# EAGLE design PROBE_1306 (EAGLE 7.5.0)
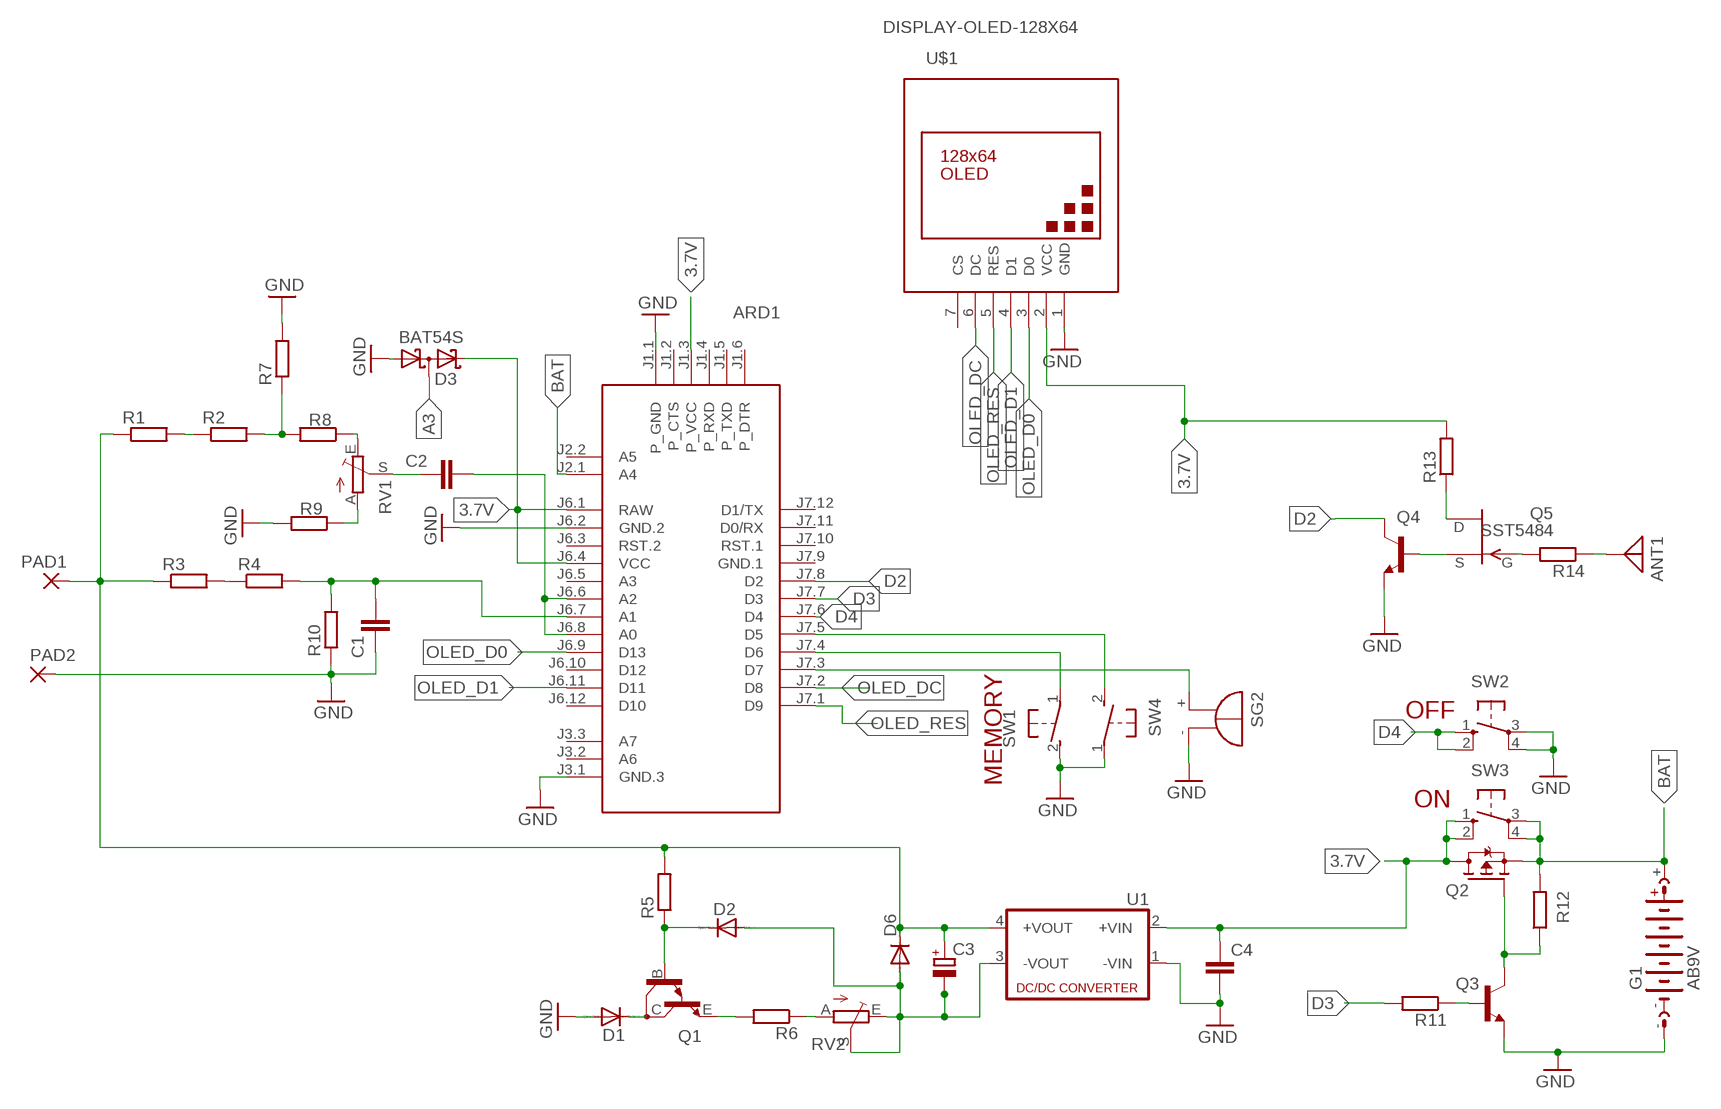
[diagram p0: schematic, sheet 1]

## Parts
ANT1  ANTENNA  [PAD-01]
ARD1  ARDUINO-PRO-MINI-3.3V  [ARDUINO-PRO-MINI]
C1  C-EUC1206  [C1206]
C2  C-EUC1206  [C1206]
C3  CPOL-EUC/6032-28R  [C/6032-28R]
C4  C-EUC1206  [C1206]
D1  CGRM4007-G  [SOD-123_MINI-SMA]
D2  CGRM4007-G  [SOD-123_MINI-SMA]
D3  BAT54S  [SOT23]
D6  CGRM4001-G  [SOD-123_MINI-SMA]
G1  AB9V  [AB9V]
PAD1  3,81/1,1  [3,81/1,1]
PAD2  3,81/1,1  [3,81/1,1]
Q1  BDV65  [SOT93]
Q2  STR2P3LLH6  [SOT23]
Q3  BC817-16LT1SMD  [SOT23-BEC]
Q4  BC817-16LT1SMD  [SOT23-BEC]
Q5  SST5484  [SOT23]
R1  R-EU_R2512  [R2512]
R2  R-EU_R2512  [R2512]
R3  R-EU_R2512  [R2512]
R4  R-EU_R2512  [R2512]
R5  R-EU_R2512  [R2512]
R6  R-EU_R2512  [R2512]
R7  R-EU_R2512  [R2512]
R8  R-EU_R0805  [R0805]
R9  R-EU_R0805  [R0805]
R10  R-EU_R2512  [R2512]
R11  R-EU_R0805  [R0805]
R12  R-EU_R0805  [R0805]
R13  R-EU_R0805  [R0805]
R14  R-EU_R0805  [R0805]
RV1  TRIM_EU-CT6  [CT6]
RV2  TRIM_EU-CT6  [CT6]
SG2  BMT1205XH7.5  [BMT1205XH7.5]
SW1  31-XX  [B3F-31XX]
SW2  10-XX  [B3F-10XX]
SW3  10-XX  [B3F-10XX]
SW4  31-XX  [B3F-31XX]
U1  NME  [NME]
U$1  DISPLAY-OLED-128X64  [DISPLAY-OLED-128X64]

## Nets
3.7V: ARD1.J1.3(P_VCC) ARD1.J6.1(RAW) ARD1.J6.4(VCC) C4.1 D3.2(C2) Q2.1(D) R13.2 SW3.1(S) SW3.2(S1) U1.2(+VIN) U$1.2(VCC)
A3: ARD1.J6.7(A1) C1.2 D3.3(C1A2) R4.2 R10.2
BAT: ARD1.J2.1(A4) G1.+ Q2.3(S) R12.2 SW3.3(P) SW3.4(P1)
D2: ARD1.J7.8(D2) Q4.C
D3: ARD1.J7.7(D3) R11.2
D4: ARD1.J7.6(D4) SW2.1(S) SW2.2(S1)
GND: ARD1.J1.1(P_GND) ARD1.J3.1(GND.3) ARD1.J6.2(GND.2) C1.1 C4.2 D1.A D3.1(A1) G1.- PAD2.1(P) Q3.E Q4.E R7.2 R9.2 R10.1 SG2.- SW1.2(S) SW2.3(P) SW2.4(P1) SW4.1(P) U1.1(-VIN) U$1.1(GND)
N$1: R2.2 R7.1 R8.2
N$2: R8.1 RV1.E
N$3: R9.1 RV1.A
N$4: ARD1.J6.6(A2) ARD1.J6.8(A0) C2.2
N$5: ANT1.1 R14.1
N$6: ARD1.J7.5(D5) SW4.2(S)
N$7: Q4.B Q5.3(S)
N$8: Q1.E R6.2
N$9: R6.1 RV2.A
N$10: C3.- D2.A D6.A RV2.E RV2.S U1.3(-VOUT)
N$11: ARD1.J7.4(D6) SW1.1(P)
N$12: D1.C Q1.C
N$13: Q5.1(G) R14.2
N$14: Q5.2(D) R13.1
N$15: ARD1.J7.3(D7) SG2.+
N$16: Q2.2(G) Q3.C R12.1
N$17: C3.+ D6.C PAD1.1(P) R1.1 R3.1 R5.2 U1.4(+VOUT)
N$18: Q3.B R11.1
N$20: D2.C Q1.B R5.1
N$23: C2.1 RV1.S
N$24: R1.2 R2.1
N$26: R3.2 R4.1
OLED_D0: ARD1.J6.9(D13) U$1.3(D0)
OLED_D1: ARD1.J6.11(D11) U$1.4(D1)
OLED_DC: ARD1.J7.2(D8) U$1.6(DC)
OLED_RES: ARD1.J7.1(D9) U$1.5(RES)
Unconnected: ARD1.J1.2(P_CTS) ARD1.J1.4(P_RXD) ARD1.J1.5(P_TXD) ARD1.J1.6(P_DTR) ARD1.J2.2(A5) ARD1.J3.2(A6) ARD1.J3.3(A7) ARD1.J6.3(RST.2) ARD1.J6.5(A3) ARD1.J6.10(D12) ARD1.J6.12(D10) ARD1.J7.10(RST.1) ARD1.J7.11(D0/RX) ARD1.J7.12(D1/TX) U$1.7(CS)

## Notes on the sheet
- OFF
- MEMORY
- ON

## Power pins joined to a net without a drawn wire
GND.1: ARD1.J7.9(GND.1)

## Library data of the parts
ANT1 = discrete:ANTENNA: Antenna
ARD1 = diy-modules:ARDUINO-PRO-MINI-*: Arduino Pro Mini and compatible devices More details available here: https://www.arduino.cc/en/Main/ArduinoBoardProMini Click here to find device on ebay.com
C1 C2 C4 = rcl:C-EU: CAPACITOR, European symbol
C3 = rcl:CPOL-EU: POLARIZED CAPACITOR, European symbol
D1 D2 D6 = diode:CGRM400*-G: Molded plasitc,JEDEC SOD-123/Mini SMA
D3 = diode:BAT54S: Schottky Diodes Pin connection corrected 2011-05-04 Source: Fairchild .. BAT54.pdf
G1 = battery:AB9V: 9-V BATTERY CLIP
PAD1 PAD2 = wirepad:3,81/1,1: THROUGH-HOLE PAD
Q1 = transistor:BDV65: NPN BIPOLAR DARLINGTON TRANSISTOR
Q2 = transistor-fet:STR2P3LLH6
Q3 Q4 = transistor-npn:BC817*: NPN Transistor
Q5 = transistor-fet:?548*: N-Channel JFETs Source: VISHAY 2N5484.pdf Compatible: TO92 2N5245 J304 J305 U310 J308 J309 J310 TO72 2N4416 2N4416A 2N3823 2N4351 3N169 3N170 3N171 MFE3002 TO18 2N3796 2N3797 MFE825 Source: Motorola European Master Guide Pacge 3-59
R1-R14 = rcl:R-EU_: RESISTOR, European symbol
RV1 RV2 = pot:TRIM_EU-: POTENTIOMETER
SG2 = buzzer:BMT1205XH7.5: MAGNETIC TRANSDUCER; OC_FARNELL: unknown; OC_NEWARK: unknown
SW1 SW4 = switch-omron:31-XX: OMRON SWITCH; MPN: B3F-3100; OC_FARNELL: 959704; OC_NEWARK: 36M3582
SW2 SW3 = switch-omron:10-XX: OMRON SWITCH; MPN: B3F-1000; OC_FARNELL: 176432; OC_NEWARK: 36M3542
U1 = dc-dc-converter:NME: DC-DC CONVERTER; MF: C & D TECHNOLOGIES, INC; MPN: NME1205D; OC_FARNELL: 1021466; OC_NEWARK: 98B8198
U$1 = diy-modules:DISPLAY-OLED-128X64: 128x64 Dot Matrix OLED Module based on SSD1306 chip Variant with SPI interface More details available here: http://www.instructables.com/id/How-to-use-OLED-display-arduino-module/ SSD1306 datasheet: https://cdn-shop.adafruit.com/datasheets/SSD1306.pdf Click here to find device on ebay.com Note: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

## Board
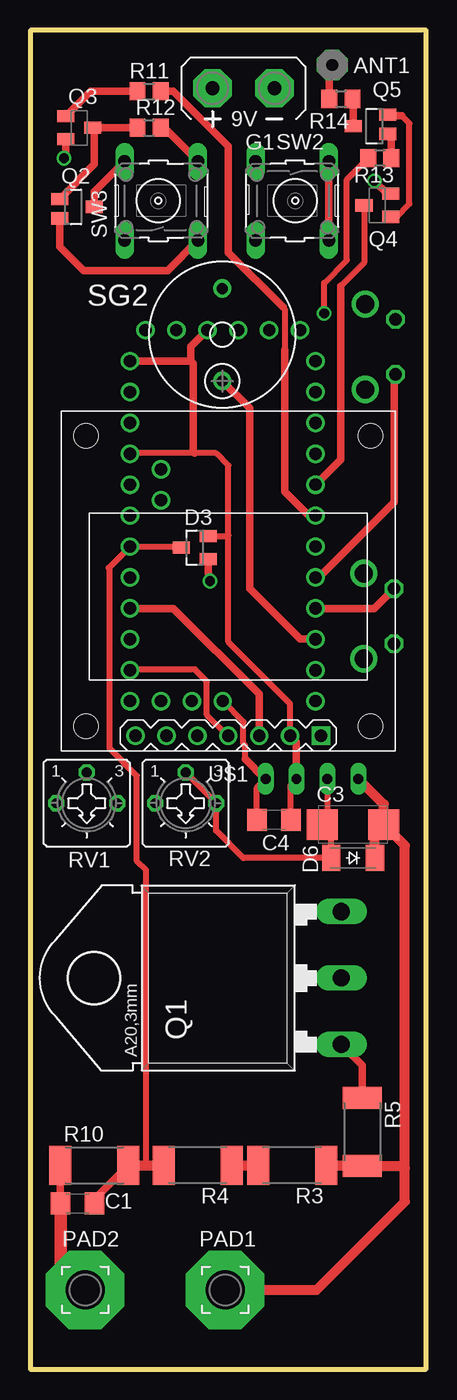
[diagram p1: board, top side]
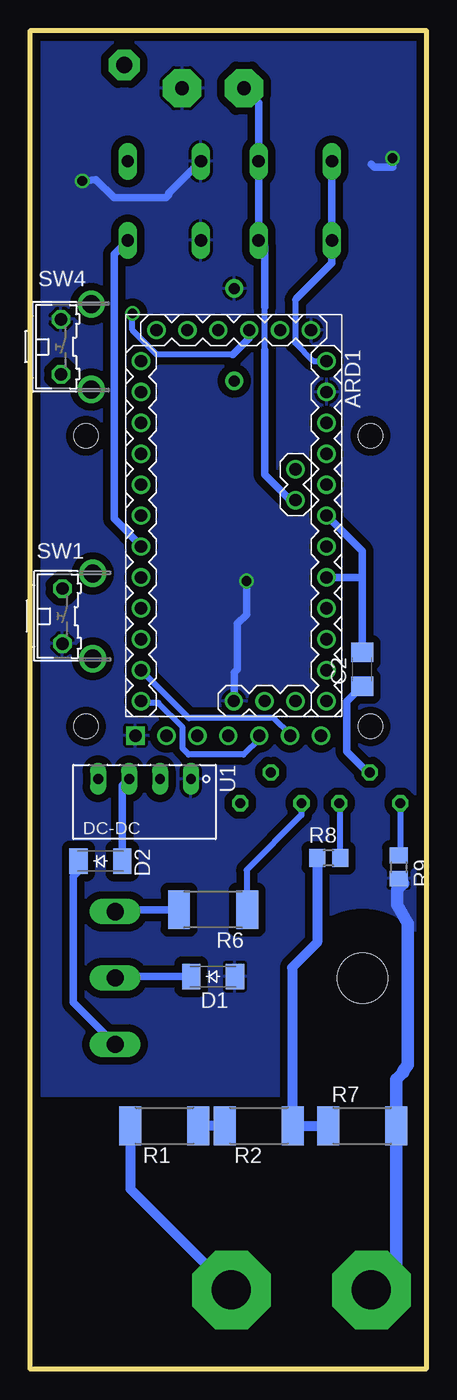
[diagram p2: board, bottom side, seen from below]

Size 32.5 x 110 mm. Coordinates in mm from the lower left corner, seen from the top.
Outline: 0,0 32.5,0 32.5,110 0,110 0,0
Copper layers (1*16): Top 0.035mm / dielectric 1.5mm / Bottom 0.035mm
Design rules "default *": minimum track width 10mil, minimum drill 24mil, track to track 8mil, track to pad 8mil, pad to pad 8mil, via to via 8mil, smd to smd 8mil, copper to edge 20mil, drill to drill 8mil, minimum pad ring 10mil, minimum via ring 8mil, stop-mask expansion 4mil, vias tented up to drill 0mil, thermal gap 10mil
bRestrict: area 0.4,22.6 to 10,28.2

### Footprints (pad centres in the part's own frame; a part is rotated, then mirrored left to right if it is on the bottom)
PAD-01 = drill 1.321 pad 2.54 octagon: 1 0,0
ARDUINO-PRO-MINI = drill 1: J1.1 -15.24,6.35; J1.2 -15.24,3.81; J1.3 -15.24,1.27; J1.4 -15.24,-1.27; J1.5 -15.24,-3.81; J1.6 -15.24,-6.35; J2.1 -1.27,5.08; J2.2 -3.81,5.08; J3.1 15.24,0; J3.2 15.24,2.54; J3.3 15.24,5.08; J6.1 -12.7,7.62; J6.2 -10.16,7.62; J6.3 -7.62,7.62; J6.4 -5.08,7.62; J6.5 -2.54,7.62; J6.6 0,7.62; J6.7 2.54,7.62; J6.8 5.08,7.62; J6.9 7.62,7.62; J6.10 10.16,7.62; J6.11 12.7,7.62; J6.12 15.24,7.62; J7.1 15.24,-7.62; J7.2 12.7,-7.62; J7.3 10.16,-7.62; J7.4 7.62,-7.62; J7.5 5.08,-7.62; J7.6 2.54,-7.62; J7.7 0,-7.62; J7.8 -2.54,-7.62; J7.9 -5.08,-7.62; J7.10 -7.62,-7.62; J7.11 -10.16,-7.62; J7.12 -12.7,-7.62
C1206 = smd 1.6 x 1.8: 1 -1.4,0; 2 1.4,0
C/6032-28R = smd 2.55 x 2.5: + 2.525,0; - -2.525,0
SOD-123_MINI-SMA = smd 1.5 x 2.1: A 1.8,0; C -1.8,0
SOT23 = smd 1 x 1.4: 1 -0.95,-1.1; 2 0.95,-1.1; 3 0,1.1
AB9V = drill 1.118 pad 3.15 octagon: + 0,2.54; - 0,-2.54
3,81/1,1 = drill 3.2 pad 6.452 octagon: 1 0,0
SOT93 = drill 1.397 long: B -5.461,-10.16; C 0,-10.16; E 5.461,-10.16 | hole 4.115: 0,10.16
SOT23' = smd 1 x 1.4: 1 0,1.735; 2 -0.632,-1.1; 3 0.95,-1.1
SOT23-BEC = smd 1 x 1.4: B -0.95,-1.1; C 0,1.1; E 0.95,-1.1
R2512 = smd 1.8 x 3.2: 1 -2.8,0; 2 2.8,0
R0805 = smd 1.3 x 1.5: 1 -0.95,0; 2 0.95,0
CT6 = drill 0.813 octagon: A 2.515,0; E -2.515,0; S 0,-2.54
BMT1205XH7.5 = drill 0.9 pad 1.5: + 3.8,0; - -3.8,0
B3F-31XX = drill 1.016 octagon: 1 -2.261,-1.245; 2 2.261,-1.245 | drill 1.499 pad 2.159: 3 -3.505,1.245; 4 3.505,1.245
B3F-10XX = drill 1.016 long: 1 -3.251,2.761; 2 3.251,2.761; 3 -3.251,-3.261; 4 3.251,-3.261
NME = drill 0.813 long: 1 0,3.81; 2 0,1.27; 3 0,-1.27; 4 0,-3.81
DISPLAY-OLED-128X64 = drill 1 square: 1 -7.62,12.7 | drill 1: 2 -5.08,12.7; 3 -2.54,12.7; 4 0,12.7; 5 2.54,12.7; 6 5.08,12.7; 7 7.62,12.7 | hole 2: -11.684,11.938; 11.684,11.938; 11.684,-11.938; -11.684,-11.938

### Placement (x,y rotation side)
ANT1  24.8,107.16 0 top
ARD1  15.8,70.13 270 bottom
C1  3.88,13.62 0 top
C2  5.25,57.5 90 bottom
C3  26.5,44.75 0 top
C4  20,45.12 180 top
D1  17.5,32.25 0 bottom
D2  26.75,41.75 0 bottom
D3  13.5,67.5 90 top
D6  26.5,42 180 top
G1  17.5,105.25 90 top
PAD1  16,6.5 0 top
PAD2  4.5,6.5 0 top
Q1  15.38,32.12 90 top
Q2  STR2P3LLH6  [SOT23']  3.5,95.5 270 top
Q3  4,102 270 top
Q4  28.5,95.62 90 top
Q5  SST5484  [SOT23']  28.25,102.12 90 top
R1  21.5,20 0 bottom
R2  13.75,20 0 bottom
R3  21.5,16.75 180 top
R4  13.75,16.75 180 top
R5  27.25,19.5 270 top
R6  17.5,37.75 180 bottom
R7  5.25,20 0 bottom
R8  8,42 180 bottom
R9  2.25,41.25 270 bottom
R10  5.25,16.75 0 top
R11  9.75,105 0 top
R12  9.75,102 0 top
R13  28.7,99.5 180 top
R14  25.5,104.38 0 top
RV1  4.62,46.5 180 top
RV2  12.75,46.5 180 top
SG2  15.75,85 270 top
SW1  28.62,61.88 270 bottom
SW2  21.75,96 270 top
SW3  10.5,96 90 top
SW4  28.75,84 270 bottom
U1  23.12,48.5 270 bottom
U$1  16.25,64.75 180 top

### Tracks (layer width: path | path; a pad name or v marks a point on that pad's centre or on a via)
3.7V  (via drill 0.8)
  Top 0.5: ARD1.J6.4 8.22,75.25 13.5,75.25 15.25,75.25 16.25,74.25 16.25,68.5 | U$1.2 21.33,54.67 16.25,59.75 16.25,68.5 | D3.2 16.2,68.45 16.25,68.5 | C4.1 21.4,48.05 U1.2 | v24.12,86.75 24.12,89.25 26,91.12 26,97.75 R13.2
  Top 0.61: U1.2 21.86,51.52 U$1.2 | ARD1.J6.1 13.17,82.83 | 13.17,82.83 13.38,82.62 13.38,75.38 13.5,75.25 | 13.17,82.83 13.17,84.01 ARD1.J1.3 | Q2.1 5.24,96.75 SW3.2
  Bottom 0.5: 10.62,88 10.75,87.88 10.75,84.33 9.25,82.83 ARD1.J6.1 | 15.88,83.38 22.12,83.38 24.12,85.38 v24.12,86.75
  Bottom 0.61: 10.62,88 7.74,90.89 SW3.1 SW3.2 | ARD1.J1.3 14.53,84.72 15.88,83.38
A3
  Top 0.5: 9.5,16.75 9.5,41 8.75,41.75 8.75,48.75 6.5,51 6.5,65.75 6.42,65.83 ARD1.J6.7 12.31,67.59 D3.3
  Top 0.61: C1.2 5.28,13.97 R10.2
  Top 0.813: R10.2 9.5,16.75 R4.2
BAT
  Top 0.61: R12.2 11.01,102 SW3.4 | Q2.3 2.4,92.22 4.38,90.25 11.26,90.25 SW3.3
  Bottom 0.5: 13.25,83.75 13.25,87.25
  Bottom 0.61: ARD1.J2.1 11.15,71.4 13.25,73.5 13.25,83.75 | 13.25,87.25 13.25,92.24 SW3.3 SW3.4 13.76,104.05 G1.+
D2
  Top 0.5: Q4.C 27.4,90.9 25.5,89
  Top 0.61: 25.5,89 25.5,74.75 ARD1.J7.8
D3
  Top 0.5: 20.75,87.25 20.88,87.12 20.88,83.75
  Top 0.61: R11.2 11.75,105 16.25,100.5 16.25,91.75 20.75,87.25 | 20.88,83.75 20.88,72.12 22.75,70.25 23.3,70.25 ARD1.J7.7
D4
  Top 0.61: SW2.2 SW2.1
  Bottom 0.61: ARD1.J7.6 23.42,67.67 25.62,69.88 25.62,91.63 SW2.2
GND  (via drill 0.8)
  Top 0.5: C4.2 18.6,47.78 U1.1 | 17.62,50.12 17.62,51.25 17.5,51.38 17.5,53.19 ARD1.J3.1
  Top 0.61: D3.1 14.6,65.4 v14.75,64.75 | R10.1 2.45,13.65 C1.1 | Q3.E 2.9,99.65 v2.75,99.5 | U1.1 19.25,48.5 17.62,50.12 | Q4.E 29.3,96.58 v28.25,97.62
  Top 1.016: C1.1 2.48,8.53 PAD2.1
  Bottom 0.61: v14.75,64.75 14.75,62 15.5,61.25 15.5,57.5 15.75,57.25 15.75,54.94 ARD1.J3.1 | v2.75,99.5 2.75,98.75 4.25,98.75 4.5,99 | v28.25,97.62 27.12,97.75 25.62,96.25 21.38,96.25 21.12,96.5 21.12,96.62 SW2.3
  Bottom 1.016: R9.2 1.88,39.92 2.38,39.42 2.38,38.12 1.5,36.62 1.5,25 1.88,24.5 1.88,24.38 2.45,23.8 R7.2 2.45,8.55 PAD2.1
  pour Bottom (isolate 0.61): 0.75,109.25 31.75,109.25 31.62,22.5 0.62,22.5
N$1
  Bottom 0.813: R7.1 R2.2 11,20.05 11,33 8.95,35.05 R8.2
N$2
  Bottom 0.5: R8.1 7.05,46.41 RV1.E
N$3
  Bottom 0.5: RV1.A 2.11,42.34 R9.1
N$4
  Bottom 0.61: C2.2 5.25,65.12 | 5.25,65.12 5.25,67.2 ARD1.J6.6 | ARD1.J6.8 5.33,65.05 5.25,65.12
N$5
  Top 0.61: R14.1 24.55,106.91 ANT1.1
N$6
  Top 0.61: ARD1.J7.5 23.68,65.05 29.88,71.25 29.88,81.62 SW4.2
N$7
  Top 0.5: 30.05,94.67 31.12,95.75 31.12,102.38 30.5,103
  Top 0.61: Q4.B 30.05,94.67 | 30.5,103 29.43,103 Q5.3
N$8
  Bottom 0.61: R6.2 25.37,37.75 Q1.E
N$9
  Bottom 0.5: RV2.A 10.23,45.52 14.75,41 14.75,37.8 R6.1
N$10
  Top 0.5: RV2.S 12.75,49.02 RV2.E 15.25,46.48 15.25,44.25 17.5,42 D6.A 24.7,44.02 C3.- 24.39,45.17 U1.3
  Bottom 0.61: D2.A 24.95,47.95 U1.3
N$11
  Top 0.61: ARD1.J7.4 28.24,62.51 SW1.1
N$12
  Bottom 0.61: D1.C 25.41,32.25 Q1.C
N$13
  Top 0.61: Q5.1 26.52,104.31 R14.2
N$14
  Top 0.61: R13.1 29.65,101.19 Q5.2
N$15
  Top 0.61: ARD1.J7.3 22.16,59.97 18,64.12 18,78.95 SG2.+
N$16
  Top 0.61: R12.1 Q3.C 5.25,101.85 5.25,99 2.4,96.15 Q2.2
N$17
  Top 0.813: PAD1.1 23.5,6.5 30.75,13.75 30.75,16.5 | 30.75,16.5 30.75,43.02 C3.+ | D6.C 28.3,44.02 C3.+ | C3.+ 29.02,46.41 U1.4 | 30.75,16.5 30.55,16.7 R5.2 27.2,16.75 R3.1
  Bottom 0.813: R1.1 24.3,14.8 PAD1.1
N$18
  Top 0.61: R11.1 4.95,105 Q3.B
N$20
  Top 0.61: R5.1 27.25,24.95 Q1.B
  Bottom 0.61: D2.C 28.55,40.95 29,40.5 29,30.13 Q1.B
N$23
  Bottom 0.61: RV1.S 4.79,49.04 6.5,50.75 6.5,54.85 C2.1
N$24
  Bottom 0.813: R2.1 R1.2
N$26
  Top 0.813: R4.1 R3.2
OLED_D0
  Top 0.61: U$1.3 18.79,55.46 11.75,62.5 ARD1.J6.9
OLED_D1
  Top 0.5: U$1.4 16.2,52.05 14.5,53.75 14.5,56.5 13.5,57.5 8.25,57.5 ARD1.J6.11
OLED_DC
  Bottom 0.5: U$1.6 11.17,52.17 12.5,53.5 19.49,53.5 ARD1.J7.2
OLED_RES
  Bottom 0.5: U$1.5 13.71,51.79 15,50.5 19.5,50.5 20,51 20,52.75 22,54.75 23.28,54.75 ARD1.J7.1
